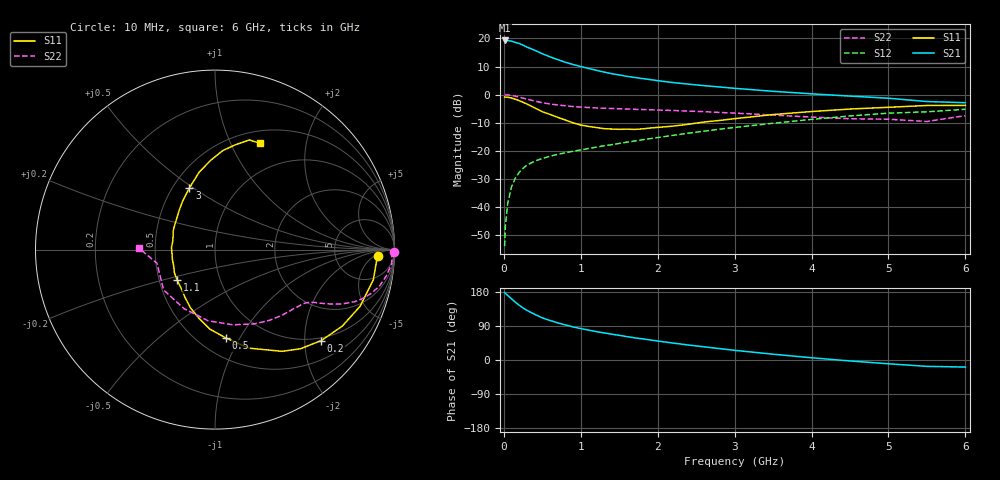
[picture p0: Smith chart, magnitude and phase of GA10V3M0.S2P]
! Infineon Technologies  Discrete & RF Semiconductors
! BF775
! Si NPN RF Bipolar Junction Transistor in SOT23
! VCE = 10 V  IC = 3 mA
! Common Emitter S-Parameters:  May  1996
# GHz  S  MA  R  50
!  f  S11  S21  S12  S22
! GHz  MAG  ANG  MAG  ANG  MAG  ANG  MAG  ANG
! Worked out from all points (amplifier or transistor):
!   36 points, 10 MHz to 6 GHz, reference 50 ohm
!   highest |S21| = 19.3 dB at 10 MHz (marker M1)
!   |S21| within 3 dB of that: start of sweep to 357.8 MHz
!   unconditionally stable (mu >= 1): 1.05 GHz to 3.076 GHz
!   at 250 MHz: K = 0.35, MSG = 21.9 dB, |S12| = -26.2 dB
!   at 1.4 GHz: K = 1.10, MAG = 10.8 dB, |S12| = -17.9 dB
!   at 6 GHz: K = 0.90, MSG = 1.2 dB, |S12| = -5.2 dB
!   S11 on the Smith chart (normalised r, x): 10 MHz: 18, -7; 200 MHz: 0.93, -2.39; 500 MHz: 0.67, -0.87; 1.1 GHz: 0.62, -0.23; 3 GHz: 0.60, +0.48; 6 GHz: 0.64, +1.30
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0.01  0.9086 -2.2  9.206 178.0  0.002 83.8  0.9968 -0.9
0.02  0.9021 -4.2  9.025 175.8  0.0046 91.2  0.9851 -1.7
0.05  0.8983 -10.7  9.163 170.5  0.0115 82.8  0.9882 -4.5
0.1  0.8681 -21.3  8.941 161.6  0.0229 78.1  0.9652 -8.8
0.15  0.8271 -31.1  8.484 152.3  0.0326 72.8  0.9379 -12.6
0.2  0.7791 -40.6  8.127 144.5  0.0412 67.9  0.9022 -15.8
0.25  0.7296 -49.2  7.582 137.3  0.0487 64.5  0.8641 -18.5
0.3  0.6789 -56.6  7.023 131.0  0.0555 62.2  0.8317 -20.4
0.4  0.5806 -71.0  6.171 120.6  0.0653 57.4  0.7691 -23.2
0.5  0.4958 -83.0  5.345 111.2  0.0729 55.2  0.7158 -25.1
0.6  0.4444 -93.6  4.704 104.3  0.0797 53.8  0.6807 -26.2
0.7  0.3936 -103.0  4.2 98.1  0.0862 52.8  0.6546 -27.1
0.8  0.3525 -112.7  3.766 92.5  0.0924 52.5  0.6323 -27.8
0.9  0.3143 -122.2  3.435 87.3  0.098 52.9  0.6134 -28.5
1.1  0.2716 -141.0  2.926 79.0  0.1096 53.8  0.5888 -30.3
1.6  0.2426 177.3  2.111 61.6  0.1423 54.9  0.5538 -35.9
2.2  0.2746 141.0  1.638 44.7  0.188 55.1  0.5213 -44.9
3  0.3726 112.5  1.294 25.5  0.26 51.2  0.469 -61.9
3.5  0.4413 101.4  1.145 15.3  0.3088 46.8  0.4311 -76.5
4.5  0.5533 85.5  0.94 -2.5  0.4174 35.6  0.3713 -117.7
5.5  0.6403 72.6  0.752 -16.8  0.4939 19.6  0.3322 -166.8
6  0.6427 67.1  0.717 -18.6  0.5482 15.1  0.4219 179.1
